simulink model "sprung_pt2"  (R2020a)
settings: Solver=ode45  StartTime=0.0  StopTime=10.0  MaxStep=0.01  RelTol=1e-3  EnableMultiTasking=on

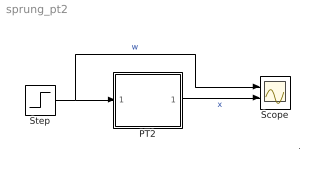
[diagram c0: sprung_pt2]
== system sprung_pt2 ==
  note: .
  PT2 : Subsystem  mask(PT2){D=0.2, om0=3, b0=1.0}
      mask prompts: D "Daempfungsgrad"; om0 "Eigenfrequenz"; b0 "Staerke"
      mask help: schwingfaehige Regelstrecke mit Daempfung D Eigenfrequenz om0 Starke b0
  Scope : Scope  NumInputPorts=2
  Step : Step  SampleTime=0
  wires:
  Step/1 -> PT2/1(u), Scope/1  "w"
  PT2/1(x) -> Scope/2  "x"

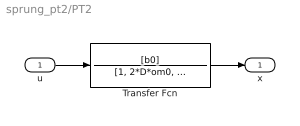
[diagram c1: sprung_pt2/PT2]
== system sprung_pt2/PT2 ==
  u : Inport
  Transfer Fcn : TransferFcn  Numerator=[b0]  Denominator=[1, 2*D*om0, om0*om0]
  x : Outport
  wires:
  Transfer Fcn/1 -> x/1
  u/1 -> Transfer Fcn/1
